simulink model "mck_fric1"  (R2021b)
settings: Solver=VariableStepAuto  StartTime=0.0  StopTime=20  RelTol=1e-3
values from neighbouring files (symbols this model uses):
  C = 1    [mck_fric.m]
  FDJ = 0.25    [mck_fric.m]
  FSJ = 0.5    [mck_fric.m]
  K = 10    [mck_fric.m]
  M = 1    [mck_fric.m]
undefined symbols (not defined in the file or in its folder): dynamics
libraries: fl_lib x9, nesl_utility x4

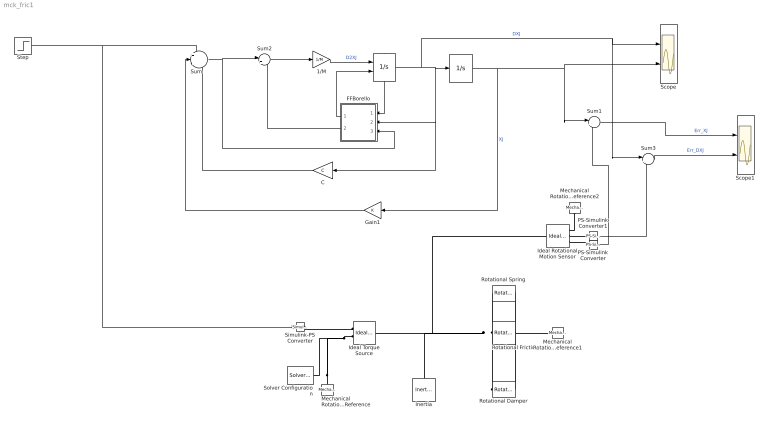
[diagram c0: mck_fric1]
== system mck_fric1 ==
  " " : Integrator  ExternalReset=rising  ShowStatePort=on
  "  " : Integrator  UpperSaturationLimit=dynamics.ThUmax/dynamics.tau  LowerSaturationLimit=dynamics.ThUmin/dynamics.tau
  1/M : Gain  Gain=1/M
  C : Gain  Gain=C
  FFBorello : Subsystem
  Gain1 : Gain  Gain=K
  Ideal Rotational Motion Sensor : fl_lib/Mechanical/Mechanical Sensors/Ideal Rotational Motion Sensor  wrap_angle=simscape.enum.onoff.off  offset=0 rad
  Ideal Torque Source : fl_lib/Mechanical/Mechanical Sources/Ideal Torque Source
  Inertia : fl_lib/Mechanical/Rotational Elements/Inertia  inertia=M kg*m^2  num_ports=foundation.enum.numPorts2.one  w_specify=off  w_priority=High  w=0 rad/s  w_nominal_specify=off  w_nominal_unit=rad/s  w_nominal_value=1  t_specify=off  t_priority=None  t=0 N*m  t_nominal_specify=off  t_nominal_unit=N*m  t_nominal_value=1
  Mechanical Rotational Reference : fl_lib/Mechanical/Rotational Elements/Mechanical Rotational Reference
  Mechanical Rotational Reference1 : fl_lib/Mechanical/Rotational Elements/Mechanical Rotational Reference
  Mechanical Rotational Reference2 : fl_lib/Mechanical/Rotational Elements/Mechanical Rotational Reference
  PS-Simulink Converter : nesl_utility/PS-Simulink Converter  PhysicalDomain=network_engine_domain  SubClassName=ps_output  LeftPortType=input  RightPortType=output  PseudoPeriodic=off  Frequencies=[]  Unit=inherit  AffineConversion=off
  PS-Simulink Converter1 : nesl_utility/PS-Simulink Converter  PhysicalDomain=network_engine_domain  SubClassName=ps_output  LeftPortType=input  RightPortType=output  PseudoPeriodic=off  Frequencies=[]  Unit=inherit  AffineConversion=off
  Rotational Damper : fl_lib/Mechanical/Rotational Elements/Rotational Damper  D=C N*m/(rad/s)  w_specify=off  w_priority=None  w=0 rad/s  w_nominal_specify=off  w_nominal_unit=rad/s  w_nominal_value=1  t_specify=off  t_priority=None  t=0 N*m  t_nominal_specify=off  t_nominal_unit=N*m  t_nominal_value=1
  Rotational Friction : fl_lib/Mechanical/Rotational Elements/Rotational Friction  brkwy_trq=FSJ N*m  brkwy_vel=0.00001201 rad/s  Col_trq=FDJ N*m  visc_coef=0 N*m/(rad/s)  w_specify=off  w_priority=None  w=0 rad/s  w_nominal_specify=off  w_nominal_unit=rad/s  w_nominal_value=1  t_specify=off  t_priority=None  t=0 N*m  t_nominal_specify=off  t_nominal_unit=N*m  t_nominal_value=1
  Rotational Spring : fl_lib/Mechanical/Rotational Elements/Rotational Spring  spr_rate=K N*m/rad  w_specify=off  w_priority=None  w=0 rad/s  w_nominal_specify=off  w_nominal_unit=rad/s  w_nominal_value=1  t_specify=off  t_priority=None  t=0 N*m  t_nominal_specify=off  t_nominal_unit=N*m  t_nominal_value=1  phi_specify=off  phi_priority=High  phi=0 rad  phi_nominal_specify=off  phi_nominal_unit=rad  phi_nominal_value=1
  Scope : Scope  NumInputPorts=2
  Scope1 : Scope  NumInputPorts=2
  Simulink-PS Converter : nesl_utility/Simulink-PS Converter  PhysicalDomain=network_engine_domain  SubClassName=ps_input  LeftPortType=input  RightPortType=output  PseudoPeriodic=off  Frequencies=[]  NoiseDistribution=none  NoiseParameters=[]  Unit=1  AffineConversion=off  FilteringAndDerivatives=provide  SimscapeFilterOrder=1  InputFilterTimeConstant=0.001  UdotUserProvided=0
  Solver Configuration : nesl_utility/Solver Configuration  PhysicalDomain=network_engine_domain  SubClassName=solver  LeftPortType=input  RightPortType=generic  Tones=[]  Harmonics=[]  SimulateNoise=off  Profile=off  UseLocalSampling=off  EnableSwitchedLinearOptims=on  FrequencyDomain=off  UseCCode=off  RelTol=0.001  AbsTol=1e-06  MinStep=1e-09  ToWorkspace=off  RevertToSquareIcSolve=off  NumHomotopyIterations=100  PhasorMode=off  PhasorModeNumHarmonics=1  DoDC=off  ResidualTolerance=1e-09  UseLocalSolver=off  LocalSolverChoice=NE_BACKWARD_EULER_ADVANCER  LocalSolverSampleTime=0.001  DoFixedCost=off  MaxNonlinIter=3  MaxModeIter=2  ComputeImpulses=off  ImpulseIterations=2  LinearAlgebra=auto  EquationFormulation=NE_TIME_EF  DelaysMemoryBudget=1024  AutomaticFiltering=on  FilteringTimeConstant=0.001  PartitionStorageMethod=AS_NEEDED  PartitionMemoryBudget=1024  PartitionMethod=ROBUST
  Step : Step  Time=10  Before=10  After=-10  SampleTime=0
  Sum : Sum  Inputs=+--
  Sum1 : Sum  Inputs=|+-
  Sum2 : Sum  Inputs=|+-
  Sum3 : Sum  Inputs=|+-
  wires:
  Sum/1 -> FFBorello/3(Act Torque), Sum2/1
  1/M/1 -> " "/1  "D2XJ"
  FFBorello/2(TF) -> Sum2/2
  Sum2/1 -> 1/M/1
  " "/1 -> Sum3/1, Scope/1, "  "/1, C/1, FFBorello/2(DXJ)  "DXJ"
  " "/State -> FFBorello/1(DXJ SP)
  C/1 -> Sum/3
  "  "/1 -> Sum1/1, Scope/2, Gain1/1  "XJ"
  Gain1/1 -> Sum/2
  PS-Simulink Converter/1 -> Sum1/2
  Sum1/1 -> Scope1/1  "Err_XJ"
  PS-Simulink Converter1/1 -> Sum3/2
  Sum3/1 -> Scope1/2  "Err_DXJ"
  Step/1 -> Simulink-PS Converter/1, Sum/1
  FFBorello/1(Reset_DXJ) -> " "/2
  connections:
  Ideal Torque Source/RConn2 -- Mechanical Rotational Reference/LConn1 -- Solver Configuration/RConn1
  Simulink-PS Converter/RConn1 -- Ideal Torque Source/RConn1
  Rotational Damper/LConn1 -- Ideal Rotational Motion Sensor/LConn1 -- Inertia/LConn1 -- Ideal Torque Source/LConn1 -- Rotational Spring/LConn1 -- Rotational Friction/LConn1
  Rotational Spring/RConn1 -- Mechanical Rotational Reference1/LConn1 -- Rotational Damper/RConn1 -- Rotational Friction/RConn1
  PS-Simulink Converter1/LConn1 -- Ideal Rotational Motion Sensor/RConn2
  Mechanical Rotational Reference2/LConn1 -- Ideal Rotational Motion Sensor/RConn1
  PS-Simulink Converter/LConn1 -- Ideal Rotational Motion Sensor/RConn3

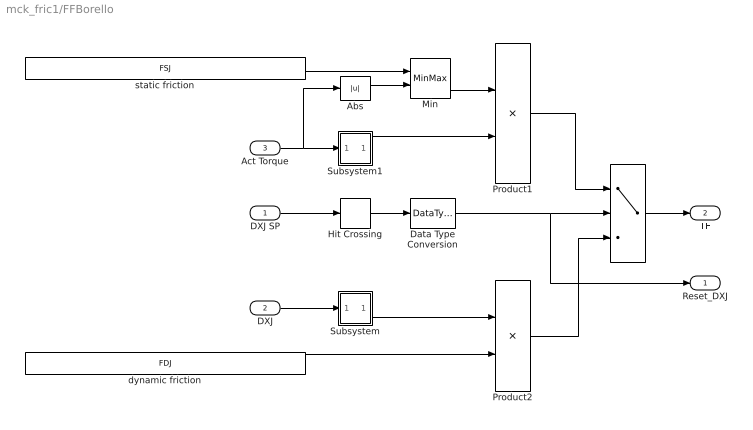
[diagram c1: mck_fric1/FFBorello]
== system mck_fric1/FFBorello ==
  DXJ SP : Inport
  DXJ : Inport  Port=2
  Act Torque : Inport  Port=3
  "   " : Switch  Threshold=0.5
  Abs : Abs
  Data Type Conversion : DataTypeConversion  OutDataTypeStr=double
  Hit Crossing : HitCross
  Min : MinMax  Inputs=2  InputSameDT=on  SaturateOnIntegerOverflow=on
  Product1 : Product  InputSameDT=on  RndMeth=Zero  SaturateOnIntegerOverflow=on
  Product2 : Product  InputSameDT=on  RndMeth=Zero  SaturateOnIntegerOverflow=on
  Subsystem : Subsystem
  Subsystem1 : Subsystem
  dynamic friction : Constant  Value=FDJ
  static friction : Constant  Value=FSJ
  Reset_DXJ : Outport
  TF : Outport  Port=2
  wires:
  Product2/1 -> "   "/3
  DXJ/1 -> Subsystem/1(In1)
  "   "/1 -> TF/1
  Product1/1 -> "   "/1
  Min/1 -> Product1/1
  Act Torque/1 -> Subsystem1/1(In1), Abs/1
  Abs/1 -> Min/2
  Hit Crossing/1 -> Data Type Conversion/1
  Subsystem/1(Out1) -> Product2/1
  Subsystem1/1(Out1) -> Product1/2
  Data Type Conversion/1 -> "   "/2, Reset_DXJ/1
  DXJ SP/1 -> Hit Crossing/1
  static friction/1 -> Min/1
  dynamic friction/1 -> Product2/2

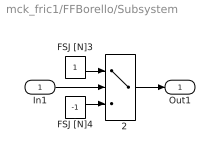
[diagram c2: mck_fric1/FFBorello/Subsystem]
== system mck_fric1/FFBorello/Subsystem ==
  In1 : Inport
  "   2" : Switch
  FSJ [N]3 : Constant
  FSJ [N]4 : Constant  Value=-1
  Out1 : Outport
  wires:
  FSJ [N]3/1 -> "   2"/1
  FSJ [N]4/1 -> "   2"/3
  In1/1 -> "   2"/2
  "   2"/1 -> Out1/1

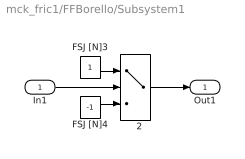
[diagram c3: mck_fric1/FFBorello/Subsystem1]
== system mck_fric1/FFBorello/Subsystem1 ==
  In1 : Inport
  "   2" : Switch
  FSJ [N]3 : Constant
  FSJ [N]4 : Constant  Value=-1
  Out1 : Outport
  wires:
  FSJ [N]3/1 -> "   2"/1
  FSJ [N]4/1 -> "   2"/3
  In1/1 -> "   2"/2
  "   2"/1 -> Out1/1
